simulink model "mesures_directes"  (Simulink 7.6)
settings: Solver=ode15s  StartTime=0.0  StopTime=0.14  RelTol=1e-3
PreLoadFcn:
  | clc
InitFcn:
  | R=1;
  | L=0.01;
  | C=1e-3;
StopFcn:
  | close all
  | load mesures_U_et_I.mat
  | plot(x(1,:),x(2,:),x(1,:),x(3,:))
  | grid
  | title('Mesure directe de la tension et du courant - Circuit RLC')
  | xlabel('temps')
libraries: powerlib x8

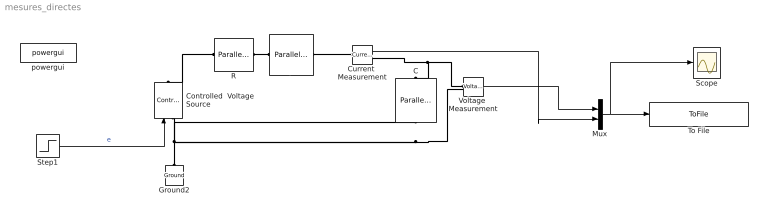
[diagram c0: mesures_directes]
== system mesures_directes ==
  C : powerlib/Elements/Parallel RLC Branch  DialogController=POWERSYS.PowerSysDialog  PhysicalDomain=powersysdomain  SubClassName=unknown  LeftPortType=p1  RightPortType=p1  LConnTagsString=a  RConnTagsString=__new0  BranchType=C  Resistance=1  Inductance=1e-3  SetiL0=off  InitialCurrent=0  Capacitance=C  Setx0=off  InitialVoltage=0  Measurements=Branch voltage and current
  Controlled  Voltage Source : powerlib/Electrical Sources/Controlled Voltage Source  DialogController=POWERSYS.PowerSysDialog  SystemSampleTime=-1  Initialize=on  Source_Type=AC  Amplitude=0  Phase=0  Frequency=0  Measurements=None
  Current  Measurement : powerlib/Measurements/Current Measurement  DialogController=POWERSYS.PowerSysDialog  SystemSampleTime=-1  PhasorSimulation=off  OutputType=Complex  PSBequivalent=0
  Ground2 : powerlib/Elements/Ground  DialogController=POWERSYS.PowerSysDialog  PhysicalDomain=powersysdomain  SubClassName=unknown  LeftPortType=p1  RightPortType=p1  LConnTagsString=a
  L : powerlib/Elements/Parallel RLC Branch  DialogController=POWERSYS.PowerSysDialog  PhysicalDomain=powersysdomain  SubClassName=unknown  LeftPortType=p1  RightPortType=p1  LConnTagsString=a  RConnTagsString=__new0  BranchType=L  Resistance=1  Inductance=L  SetiL0=off  InitialCurrent=0  Capacitance=1e-6  Setx0=off  InitialVoltage=0  Measurements=None
  Mux : Mux  Inputs=2
  R : powerlib/Elements/Parallel RLC Branch  DialogController=POWERSYS.PowerSysDialog  PhysicalDomain=powersysdomain  SubClassName=unknown  LeftPortType=p1  RightPortType=p1  LConnTagsString=a  RConnTagsString=__new0  BranchType=R  Resistance=R  Inductance=10e-03  SetiL0=off  InitialCurrent=0  Capacitance=[]  Setx0=off  InitialVoltage=0  Measurements=None
  Scope : Scope
  Step1 : Step  Time=0.02  SampleTime=0
  To File : ToFile  Filename=mesures_U_et_I  MatrixName=x
  Voltage  Measurement : powerlib/Measurements/Voltage Measurement  DialogController=POWERSYS.PowerSysDialog  SystemSampleTime=-1  PhasorSimulation=off  OutputType=Complex  PSBequivalent=0
  powergui : powerlib/powergui  SystemSampleTime=-1  SimulationMode=Continuous  SampleTime=0  frequency=60  SPID=off  DisableSnubberDevices=off  DisableRonSwitches=off  DisableVfSwitches=off  SwTol=0  Interpol=off  frequencyindice=0  echomessages=off  HookPort=off  DisplayEquations=off  FunctionMessages=off  EnableUseOfTLC=off  x0status=blocks  RestoreLinks=warning  ResistiveCurrentMeasurement=off  Frange=[0:2:500]  Ylog=off  Xlog=on  ShowGrid=on  save=off  variable=ZData  ZoomFFT=on  StartTime=0.0  cycles=1  DisplayStyle=1  fundamental=60  FreqAxis=off  MaxFrequency=1000  frequencyindicesteady=60  RmsSteady=1  display=off  Ts=0  methode=off
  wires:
  Step1/1 -> Controlled  Voltage Source/1  "e"
  Mux/1 -> To File/1, Scope/1
  Current  Measurement/1 -> Mux/2
  Voltage  Measurement/1 -> Mux/1
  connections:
  R/RConn1 -- Controlled  Voltage Source/RConn1
  R/LConn1 -- L/LConn1
  Voltage  Measurement/LConn1 -- C/LConn1 -- Current  Measurement/RConn1
  Voltage  Measurement/LConn2 -- C/RConn1 -- Ground2/LConn1 -- Controlled  Voltage Source/LConn1
  L/RConn1 -- Current  Measurement/LConn1
